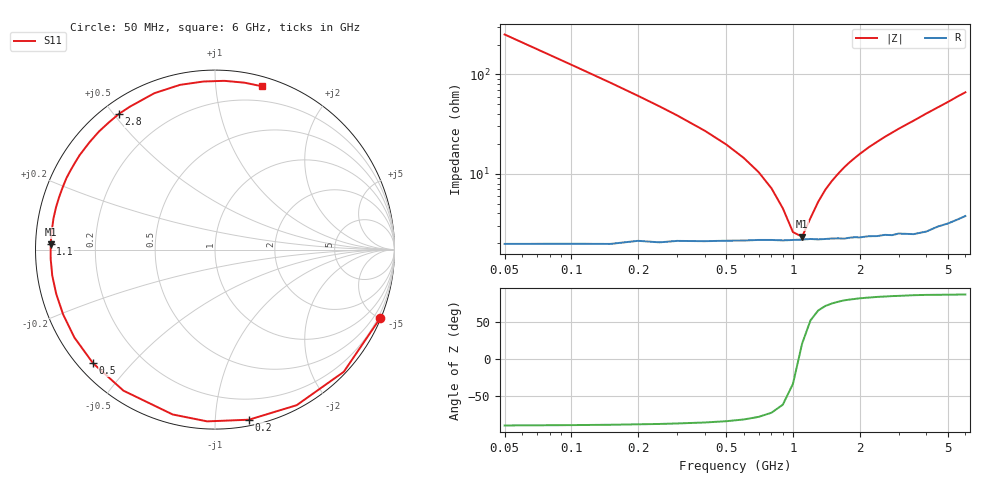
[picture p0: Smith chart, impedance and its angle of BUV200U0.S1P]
! Infineon Technologies  Discrete & RF Semiconductors
! BB 833
! Si Tuning Diode in SOD323
! VR = 0.2 V
! S-Parameters:  June  1999
# GHz  S  MA  R  50
!  f  S11
! GHz  MAG  ANG
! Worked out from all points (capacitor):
!   34 points, 50 MHz to 6 GHz, reference 50 ohm
!   read as one part to ground: C = 12.6 pF near 50 MHz
!   lowest |Z| = 2.34 ohm at 1.1 GHz (marker M1)
!   series resonance near 1.063 GHz, so ESL is about 1.8 nH
!   S11 on the Smith chart (normalised r, x): 50 MHz: 0.04, -5.05; 200 MHz: 0.04, -1.22; 500 MHz: 0.04, -0.39; 1.1 GHz: 0.04, +0.02; 2.8 GHz: 0.05, +0.52; 6 GHz: 0.08, +1.32
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0.05  0.997 -22.4
0.1  0.9892 -43.5
0.15  0.9791 -62.3
0.2  0.9664 -78.7
0.25  0.958 -92.6
0.3  0.9484 -104.4
0.4  0.937 -123.0
0.5  0.9289 -137.0
0.6  0.9239 -148.0
0.7  0.9201 -156.9
0.8  0.9184 -164.4
0.9  0.9182 -170.9
1.1  0.9163 178.1
1.3  0.9166 169.1
1.4  0.9165 165.0
1.6  0.9169 157.8
1.8  0.9179 151.1
2  0.9196 145.1
2.2  0.9201 139.5
2.4  0.9225 134.5
2.8  0.9264 125.2
3  0.9268 120.8
3.5  0.9346 111.2
4  0.9383 102.0
4.5  0.9387 94.0
5  0.9418 86.8
5.5  0.9444 79.9
6  0.9466 74.1
